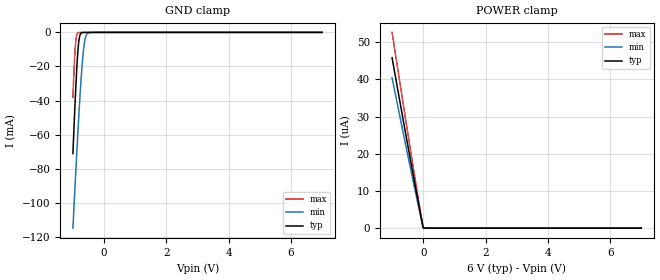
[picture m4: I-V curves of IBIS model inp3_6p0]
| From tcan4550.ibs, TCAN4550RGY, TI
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|   inp3_6p0 Model
[Model]   inp3_6p0
Model_type   Input
Vinl = 3
Vinh = 4
|   typ   min   max
C_comp   2.765pF   2.714pF   2.777pF
|  Where Nom  PVT is Nominal Process, 6V,   27C
|   Fast PVT is Strong Process,  6.5V, -40C
|   Slow PVT is Weak Process,   5.5V, 150C
[Model spec]
|subparameter
Vinl   3   2.5   3.5
Vinh   4   3.5   4.5
[Voltage Range]   6   5.5   6.5
|Junction Temperature
[Temperature Range]   27   150   -40
[Power Clamp Reference]   6   5.5   6.5
[GND Clamp Reference]   0   0   0
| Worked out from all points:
|   GND clamp passes 1 mA (typ) near -0.76 V on its own axis
[GND Clamp]
|   Voltage   I(typ)   I(min)   I(max)
-1V       -71.04mA   -114.8mA   -38.01mA
-952mV    -50.3mA    -97.45mA   -17.57mA
-912mV    -34.17mA   -83.26mA   -5.975mA
-888mV    -25.37mA   -74.9mA    -2.441mA
-856mV    -15.22mA   -63.98mA   -624uA
-808mV    -4.988mA   -48.28mA   -102uA
-776mV    -1.851mA   -38.44mA   -54.21uA
-728mV    -357.2uA   -25.03mA   -40.31uA
-664mV    -59.88uA   -11.04mA   -35.62uA
-600mV    -30.43uA   -3.262mA   -32.07uA
-528mV    -24.64uA   -571.1uA   -28.17uA
7V        0A         0A         0A
[POWER Clamp]
|   Voltage   I(typ)   I(min)   I(max)
-1V       45.82uA    40.45uA    52.66uA
-552mV    24.85uA    21.88uA    28.53uA
-200mV    8.752uA    7.732uA    10.03uA
-8mV      299.8nA    265.4nA    345.2nA
16mV      0A         0A         0A
7V        0A         0A         0A
